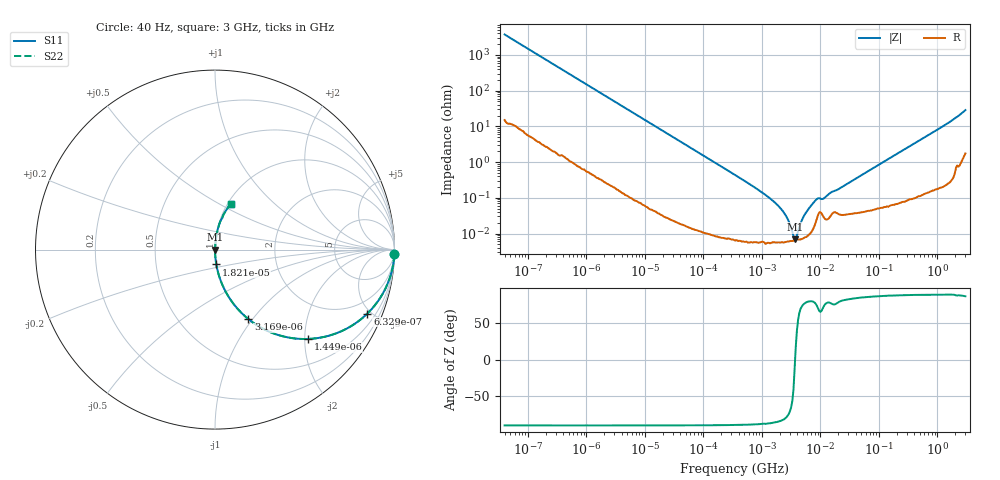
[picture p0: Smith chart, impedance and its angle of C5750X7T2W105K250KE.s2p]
! S-parameter Generated by TDK Corporation
! Copyright(C) 2015 TDK Corporation.
! All Rights Reserved.
! TDK P/N: C5750X7T2W105K250KE (Multilayer Ceramic Chip Capacitors)
! Property: C=1uF
! Size(LxWxT): 5.7x5x2.5mm, 0.224x0.197x0.098inches
! Model Type: s2p (Touchstone File Format Version 1.0)
! Frequency: DC=Yes Start=0.00004MHz Stop=3000MHz 396points Log-sweep
! Note: This model was converted from impedance.
! Model Generated on Jun. 23, 2015
! Hash(MD5):
! Port Assignments:
!  1 ---| |--- 2
! Applicable Conditions:
!  Temperature = 25 degC
!  DC Bias Voltage = 0 V
!  Small Signal Operation
! Terms and conditions regarding TDK Simulation Models
! (1)This simulation model is being provided solely for informational purposes. Please refer to the specifications of the products in terms of detailed characteristics of such products.
! (2)In no event shall TDK Corporation of any of its subsidiaries be liable for any loss or damage arising, directly or indirectly,
!  From any information contained in this simulation model, including, but not limited to loss or damages arising from any inaccuracies, omissions or errors in connection with such information.
! (3)Any and all copyrights on this simulation model are owned by TDK Corporation.
!  Duplication or redistribution of this simulation model without prior written permission from TDK Corporation is prohibited.
! (4)This simulation model is subject to any modification or change without any prior notice.
! (5)Neither TDK Corporation nor any of its subsidiaries shall make any warranty, express or implied,
!  Including but not limited to the correctness, implied warranties of merchantability and fitness for a particular purpose with respect to this simulation models.
! (6)The use of this simulation model shall be deemed to have consented to the terms and conditions hereof.
# MHz S MA R 50
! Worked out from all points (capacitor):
!   395 points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, 40 Hz to 3 GHz, reference 50 ohm
!   read as one part in series: C = 1.06 uF near 41.88 Hz
!   lowest |Z| = 6.94 mohm at 3.622 MHz (marker M1)
!   series resonance near 3.692 MHz, so ESL is about 1.7 nH
!   S11 on the Smith chart (normalised r, x): 40 Hz: 1, -75; 632.9 Hz: 1.02, -4.75; 1.449 kHz: 1.01, -2.08; 3.169 kHz: 1.00, -0.95; 18.21 kHz: 1.00, -0.17; 3 GHz: 1.03, +0.57
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4e-05  0.9995 -1.5  0.02662 88.2  0.02662 88.2  0.9995 -1.5
0.0001912643  0.9915 -7.3  0.1264 82.5  0.1264 82.5  0.9915 -7.3
0.0006328604  0.9206 -22.8  0.3872 67.0  0.3872 67.0  0.9206 -22.8
0.000834128  0.8733 -28.9  0.484 60.8  0.484 60.8  0.8733 -28.9
0.001449046  0.7196 -43.8  0.6918 46.0  0.6918 46.0  0.7196 -43.8
0.003168613  0.4296 -64.3  0.9014 25.4  0.9014 25.4  0.4296 -64.3
0.006319477  0.2327 -76.3  0.9717 13.5  0.9717 13.5  0.2327 -76.3
0.01739424  0.08687 -84.8  0.9959 5.0  0.9959 5.0  0.08687 -84.8
0.01821348  0.08299 -85.0  0.9962 4.8  0.9962 4.8  0.08299 -85.0
0.3464102  0.004379 -88.9  0.9999 0.3  0.9999 0.3  0.004379 -88.9
1.816098  0.0006436 -85.0  0.9999 0.0  0.9999 0.0  0.0006436 -85.0
2.624455  0.0002958 -78.5  0.9999 0.0  0.9999 0.0  0.0002958 -78.5
3.303516  0.0001126 -56.6  0.9999 0.0  0.9999 0.0  0.0001126 -56.6
3.622024  6.942e-05 -12.7  0.9999 0.0  0.9999 0.0  6.942e-05 -12.7
3.971241  9.056e-05 40.9  0.9999 -0.0  0.9999 -0.0  9.056e-05 40.9
5.234209  0.0003135 76.1  0.9999 -0.0  0.9999 -0.0  0.0003135 76.1
7.22376  0.0006588 79.5  0.9999 -0.0  0.9999 -0.0  0.0006588 79.5
9.092863  0.0009675 70.0  0.9997 -0.1  0.9997 -0.1  0.0009675 70.0
11.44558  0.0009645 73.1  0.9997 -0.1  0.9997 -0.1  0.0009645 73.1
150.6385  0.01269 86.6  0.9993 -0.7  0.9993 -0.7  0.01269 86.6
1040.901  0.08422 83.9  0.9946 -4.8  0.9946 -4.8  0.08422 83.9
3000  0.2711 70.8  0.9462 -15.7  0.9462 -15.7  0.2711 70.8
